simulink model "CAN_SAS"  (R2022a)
settings: Solver=FixedStepAuto  StartTime=0.0  StopTime=50  RelTol=1e-3
undefined symbols (not defined in the file): bit, canChannel, Channel, Extended, identifier, MathWorks, Virtual
libraries: canlib x2, slrealtimeutilitieslib x1, canmsglib x1

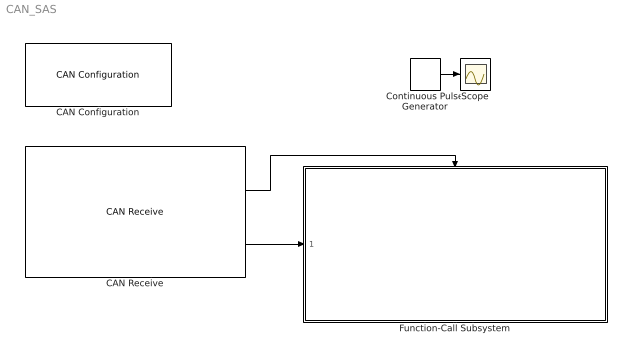
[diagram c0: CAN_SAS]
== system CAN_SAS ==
  CAN Configuration : canlib/CAN Configuration  BlockHandle=856.0001  Device=MathWorks Virtual 1 (Channel 1)  DeviceMenu=MathWorks Virtual 1 (Channel 1)  ObjConstructor=canChannel('MathWorks', 'Virtual 1', 1)  BusSpeed=500000  EnableBitParameters=off  AckMode=Normal
  CAN Receive : canlib/CAN Receive  BlockHandle=857.0001  Device=MathWorks Virtual 1 (Channel 1)  DeviceMenu=MathWorks Virtual 1 (Channel 1)  ObjConstructor=canChannel('MathWorks', 'Virtual 1', 1)  EnableStandardIDsFilter=off  StdIDsCombo=Allow all  StandardIDs=0  EnableExtendedIDsFilter=off  ExtIDsCombo=Allow only  ExtendedIDs=0x1A2402A  SampleTime=0.01  MsgsPerTimestep=all  InternalFilterUpdateStatus=on  BusOutput=off
  Continuous Pulse Generator : DiscretePulseGenerator  PulseType=Time based  Period=1  PulseWidth=50
  Function-Call Subsystem : Subsystem  TreatAsAtomicUnit=on
  Scope : Scope
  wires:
  CAN Receive/1 -> Function-Call Subsystem/Trigger
  CAN Receive/2 -> Function-Call Subsystem/1(In1)
  Continuous Pulse Generator/1 -> Scope/1

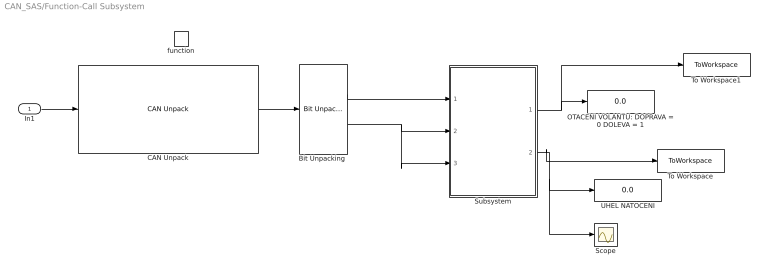
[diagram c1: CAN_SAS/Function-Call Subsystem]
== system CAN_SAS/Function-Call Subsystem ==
  In1 : Inport
  function : TriggerPort  TriggerType=function-call  VariantControl=(inherit)
  "Bit Unpacking " : slrealtimeutilitieslib/Bit Unpacking  SignExtend=off
  CAN Unpack : canmsglib/CAN Unpack  MsgList=(none)  MsgName=CAN Msg  MsgIDType=Extended (29-bit identifier)  MsgIdentifier=0x1A2402A  MsgLength=8  SignalInfo={}  IDPort=off  TimestampPort=off  ErrorPort=off  RemotePort=off  LengthPort=off  StatusPort=off  ApplyMinMax=off
  OTACENI VOLANTU: DOPRAVA = 0 DOLEVA = 1 : Display
  Scope : Scope
  Subsystem : Subsystem
  To Workspace : ToWorkspace  VariableName=uhel  SampleTime=-1
  To Workspace1 : ToWorkspace  VariableName=strana  SampleTime=-1
  UHEL NATOCENI : Display
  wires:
  In1/1 -> CAN Unpack/1
  CAN Unpack/1 -> "Bit Unpacking "/1
  Subsystem/1(Out1) -> To Workspace1/1, OTACENI VOLANTU: DOPRAVA = 0 DOLEVA = 1/1
  Subsystem/2(Out2) -> To Workspace/1, Scope/1, UHEL NATOCENI/1
  "Bit Unpacking "/1 -> Subsystem/1(In1)
  "Bit Unpacking "/2 -> Subsystem/3(In3), Subsystem/2(In2)

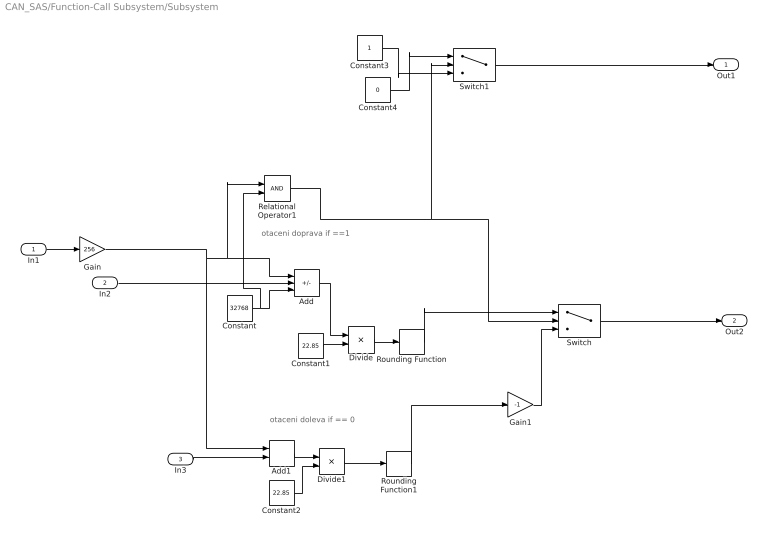
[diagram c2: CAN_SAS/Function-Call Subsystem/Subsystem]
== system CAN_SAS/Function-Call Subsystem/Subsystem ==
  note: otaceni doprava if ==1
  note: otaceni doleva if == 0
  In1 : Inport
  In2 : Inport  Port=2
  In3 : Inport  Port=3
  Add : Sum  Inputs=++-
  Add1 : Sum
  Constant : Constant  Value=32768
  Constant1 : Constant  Value=22.85
  Constant2 : Constant  Value=22.85
  Constant3 : Constant
  Constant4 : Constant  Value=0
  Divide : Product  Inputs=*/
  Divide1 : Product  Inputs=*/
  Gain : Gain  Gain=256
  Gain1 : Gain  Gain=-1
  Relational Operator1 : RelationalOperator  OutDataTypeStr=boolean  RndMeth=Simplest
  Rounding Function : Rounding
  Rounding Function1 : Rounding
  Switch : Switch  Criteria=u2 > Threshold
  Switch1 : Switch  Criteria=u2 > Threshold
  Out1 : Outport
  Out2 : Outport  Port=2
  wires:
  In2/1 -> Add/2
  Divide/1 -> Rounding Function/1
  Rounding Function/1 -> Switch/1
  Constant1/1 -> Divide/2
  In1/1 -> Gain/1
  Constant2/1 -> Divide1/2
  Relational Operator1/1 -> Switch/2, Switch1/2
  Add/1 -> Divide/1
  Constant/1 -> Relational Operator1/2, Add/3
  Rounding Function1/1 -> Gain1/1
  Gain/1 -> Add1/1, Relational Operator1/1, Add/1
  Divide1/1 -> Rounding Function1/1
  Switch1/1 -> Out1/1
  Add1/1 -> Divide1/1
  In3/1 -> Add1/2
  Switch/1 -> Out2/1
  Gain1/1 -> Switch/3
  Constant4/1 -> Switch1/1
  Constant3/1 -> Switch1/3
